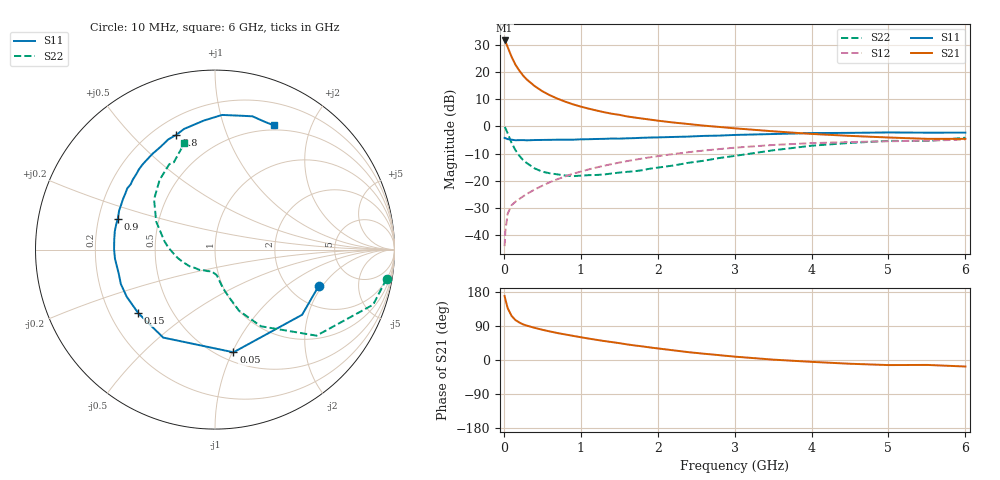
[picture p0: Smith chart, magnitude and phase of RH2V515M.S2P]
! SIEMENS Small Signal Semiconductors
! BFR106
! Si NPN RF Bipolar Junction Transistor in SOT23
! VCE = 2.5 V  IC = 15 mA
! Common Emitter S-Parameters:  August  1996
# GHz  S  MA  R  50
!  f  S11  S21  S12  S22
! GHz  MAG  ANG  MAG  ANG  MAG  ANG  MAG  ANG
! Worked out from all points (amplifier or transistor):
!   36 points, 10 MHz to 6 GHz, reference 50 ohm
!   highest |S21| = 31.5 dB at 10 MHz (marker M1)
!   |S21| within 3 dB of that: start of sweep to 57.92 MHz
!   unconditionally stable (mu >= 1): 402.5 MHz to 2.348 GHz; 5.133 GHz to end of sweep
!   at 250 MHz: K = 0.83, MSG = 22.2 dB, |S12| = -25.7 dB
!   at 1.4 GHz: K = 1.08, MAG = 7.5 dB, |S12| = -13.9 dB
!   at 6 GHz: K = 1.01, MAG = -0.5 dB, |S12| = -4.9 dB
!   S11 on the Smith chart (normalised r, x): 10 MHz: 2.87, -1.84; 50 MHz: 0.58, -1.01; 150 MHz: 0.32, -0.33; 900 MHz: 0.28, +0.14; 2.8 GHz: 0.29, +0.68; 6 GHz: 0.44, +1.49
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0.01  0.6127 -19.1  37.69 168.9  0.0063 82.0  0.9694 -9.7
0.02  0.6062 -36.8  36 159.8  0.012 75.7  0.9331 -19.2
0.05  0.5813 -79.8  28.45 136.8  0.0249 59.4  0.7414 -40.3
0.1  0.5689 -120.5  18.98 116.6  0.0355 50.3  0.4986 -59.0
0.15  0.5551 -140.5  13.61 105.5  0.0412 48.6  0.3668 -68.5
0.2  0.5576 -151.9  10.59 99.1  0.0462 50.3  0.2902 -72.6
0.25  0.5585 -159.9  8.548 94.0  0.0516 52.5  0.2396 -76.4
0.3  0.5529 -165.8  7.2 90.6  0.0574 54.7  0.2108 -78.9
0.4  0.5596 -174.7  5.486 84.9  0.069 58.1  0.169 -82.6
0.5  0.5623 179.8  4.408 79.8  0.0811 60.4  0.1467 -85.3
0.6  0.5642 174.2  3.708 75.3  0.0944 61.6  0.1371 -88.6
0.7  0.5676 169.5  3.209 71.0  0.1073 62.2  0.1309 -92.8
0.9  0.5683 162.3  2.53 63.7  0.1345 62.3  0.1215 -100.0
1.1  0.5794 154.6  2.115 56.6  0.1612 61.5  0.1268 -109.1
1.3  0.5888 148.1  1.819 50.2  0.1887 59.8  0.1303 -117.5
1.6  0.6016 139.5  1.52 41.2  0.2295 56.7  0.1458 -131.6
2.2  0.6373 123.1  1.175 25.6  0.3095 49.0  0.1904 -158.2
2.8  0.675 108.6  0.973 12.8  0.382 39.8  0.2616 177.1
3.5  0.7218 94.9  0.81 1.0  0.4542 28.7  0.3625 154.6
4.5  0.758 80.0  0.667 -9.9  0.5139 13.0  0.4959 128.5
5.5  0.7641 68.7  0.589 -13.0  0.5438 3.1  0.5375 115.3
6  0.7659 64.6  0.588 -17.2  0.5719 -4.2  0.6164 106.1
